(* FB_CylinderTemp	- number of control signals控制信号数量:
							one direction is controllable一个方向是可控的
					- type of feedback signal反馈信号的类型:
							feedback in base and work position基准和工作位置的反馈
					- with temperature signal带温度信号					*)

FUNCTION_BLOCK FB_CylinderTemp EXTENDS FB_Cylinder
VAR_INPUT
	fTempCurrent	AT %I*	: LREAL;				// Hardware input signal: cylinder temperature硬件输入信号：气缸温度
END_VAR

// =========================================================
;
// =========================================================

END_FUNCTION_BLOCK
